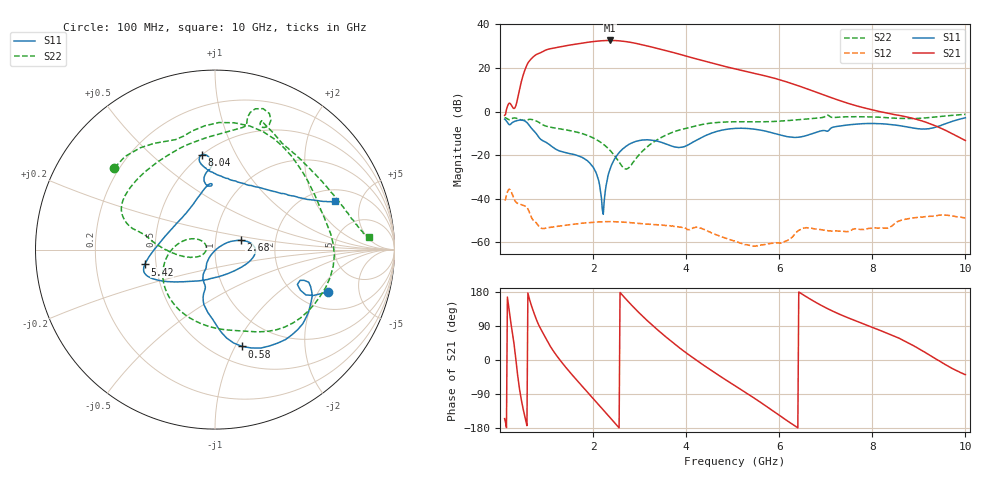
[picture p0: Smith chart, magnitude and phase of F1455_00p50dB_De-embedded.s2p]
! Integrated Device Technology
! Corporate Headquarters
! 6024 Silver Creek Valley Road
! San Jose, CA 95138  USA
! Phone:  1-408-284-8200
! Toll Free:  1-800-223-1366
! Webpage:  http://www.idt.com/
! Timing and RF Division
! 515 Groton Road, Suite 102
! Westford, MA 01886-6024
! Device:  F1455
! Description: 6-bit 0.5 dB Transmit Variable Gain Amplifier
! Frequency:  1400.0 -  2300.00 MHz
! Package:  6x6 mm Thin QFN Plastic Package: 28 pin
! State:  1
! Atten State:  0.5 dB
! Voltage:  +5.00 Volts
! Current:  213.752 mA
! Data:  The device was measured on a the F1455 evaluation board which has
!  individual transmission lines to the RF pins.  Data was collected
!  using a calibrated network analyzer.  The evaluation board was
!  de-embedded using a TRL calibration technique.
!  The reference plane is the edge of the package pin.
!  Pin  1 = CSb
!  Pin  2 = DATA
!  Pin  3 = CLK
!  Pin  4 = RSET
!  Pin  5 = GND
!  Pin  6 = RFIN  = Port 1
!  Pin  7 = GND
!  Pin  8 = NC
!  Pin  9 = NC
!  Pin 10 = NC
!  Pin 11 = NC
!  Pin 12 = NC
!  Pin 13 = NC
!  Pin 14 = /STBY
!  Pin 15 = GND
!  Pin 16 = RFOUT  = Port 2
!  Pin 17 = GND
!  Pin 18 = NC
!  Pin 19 = NC
!  Pin 20 = NC
!  Pin 21 = GND
!  Pin 22 = NC
!  Pin 23 = GND
!  Pin 24 = NC
!  Pin 25 = NC
!  Pin 26 = NC
!  Pin 27 = GND
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# GHz S dB R 50
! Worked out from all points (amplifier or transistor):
!   496 points, 100 MHz to 10 GHz, reference 50 ohm
!   highest |S21| = 32.6 dB at 2.36 GHz (marker M1)
!   |S21| within 3 dB of that: 1.272 GHz to 3.258 GHz (1.985 GHz wide, 87.7 % of centre)
!   unconditionally stable (mu >= 1): start of sweep to end of sweep
!   at 1.74 GHz: K = 4.46, MAG = 31.8 dB, |S12| = -51.2 dB
!   at 5.06 GHz: K = 27.61, MAG = 22.1 dB, |S12| = -59.6 dB
!   at 10 GHz: K = 77.25, MAG = -4.1 dB, |S12| = -48.8 dB
!   S11 on the Smith chart (normalised r, x): 100 MHz: 2.83, -2.43; 580 MHz: 0.68, -1.07; 2.68 GHz: 1.32, +0.14; 5.42 GHz: 0.43, -0.09; 8.04 GHz: 0.50, +0.74; 10 GHz: 2.64, +2.96
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0.1  -3.46 -20.6  -1.72 -154.7  -40.74 39.1  -2.82 140.8
0.4  -3.97 -36.9  8.17 -59.3  -42.24 -109.3  -3.44 50.6
0.58  -5.03 -74.3  21.39 -173.3  -44.05 -171.6  -3.88 12.4
0.78  -10.11 -101.5  26.16 107.6  -51.02 141.0  -4.29 -38.6
0.98  -13.97 -107.1  28.19 58.2  -53.50 124.3  -6.60 -74.8
1.16  -16.66 -115.6  29.16 21.5  -52.90 102.4  -7.47 -98.4
1.34  -18.43 -115.7  29.90 -8.1  -52.37 83.7  -8.11 -118.9
1.54  -19.43 -117.3  30.65 -37.6  -51.76 66.4  -8.88 -138.3
1.76  -20.93 -121.1  31.40 -68.3  -51.21 50.0  -10.04 -157.4
2.06  -27.77 -126.4  32.25 -109.3  -50.66 30.5  -12.71 177.4
2.36  -26.69 32.3  32.62 -151.2  -50.47 12.1  -17.66 152.5
2.68  -16.39 19.8  32.18 164.4  -50.75 -6.2  -26.17 166.7
3.02  -13.19 4.4  30.83 120.9  -51.37 -21.9  -19.03 -158.5
3.4  -13.66 -16.8  28.87 78.2  -51.99 -36.3  -12.67 -175.1
3.96  -16.09 -91.9  25.69 22.4  -53.14 -60.5  -7.90 167.9
4.48  -10.43 -143.3  22.68 -22.6  -55.03 -84.9  -5.43 161.3
5.06  -7.70 -160.5  19.53 -68.7  -59.55 -92.0  -4.67 148.6
5.42  -7.95 -168.0  17.77 -97.1  -61.55 -85.3  -4.68 135.6
6.7  -10.18 107.1  9.65 158.2  -53.54 -120.9  -3.21 78.2
8.04  -5.47 97.8  0.58 84.3  -53.43 -179.1  -2.48 68.4
8.36  -5.86 99.9  -0.93 68.7  -53.23 -178.4  -2.83 62.5
10  -2.83 21.9  -13.26 -38.5  -48.76 93.0  -1.29 4.6
